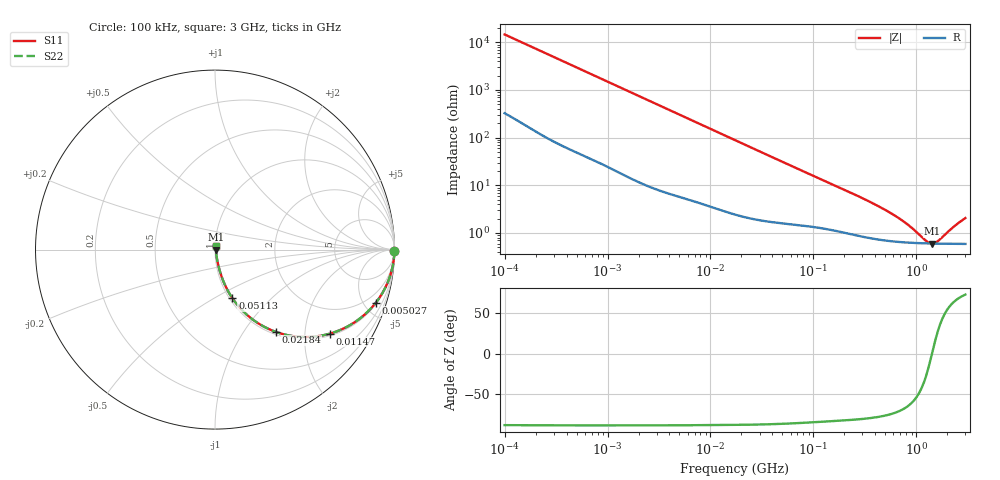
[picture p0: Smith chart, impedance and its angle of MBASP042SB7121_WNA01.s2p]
! MBASP042SB7121_WNA01  S-PARAMETER MODEL  ( Standard Model )
! Model Generated by TAIYO YUDEN Corporation (https://www.yuden.co.jp/en/)
! Version 1.0
! TAIYO YUDEN Control No. 250312
! Copyright(c) 2025 TAIYO YUDEN CO.,LTD. All Rights Reserved.
! Product Description (link to TY-COMPAS)
! https://ds.yuden.co.jp/TYCOMPAS/or/detail?pn=MBASP042SB7121KWNA01&u=M
! Products Name : Multilayer Ceramic Capacitors
! Characteristics :
!  Capacitance : 120 [pF] , Rated Voltage : 2.5 [V] , TCC : X7R
!  Case Size : 0.4 x 0.2 / 0.016 x 0.008 [mm/inch] , Thickness : 0.2 / 0.008 [mm/inch]
!  (Conditions: Temperature = 25 [degC] , DC Bias Voltage = 0 [V])
! External Node Assignments :
!  1  o---| |---o  2
! GND o---------o GND
! Frequency Range : 100kHz  -  3GHz  [ 401 STEP ]
# MHZ S RI R 50
! Freq[MHz].  S11 Real  S11 Imag  S21 Real  S21 Imag  S12 Real  S12 Imag  S22 Real  S22 Imag
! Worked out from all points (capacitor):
!   401 points, 100 kHz to 3 GHz, reference 50 ohm
!   read as one part in series: C = 108 pF near 105.3 kHz
!   lowest |Z| = 602 mohm at 1.421 GHz (marker M1)
!   series resonance near 1.421 GHz, so ESL is about 120 pH
!   S11 on the Smith chart (normalised r, x): 100 kHz: open; 5.027 MHz: 1.11, -6.04; 11.47 MHz: 1.06, -2.67; 21.84 MHz: 1.04, -1.41; 51.13 MHz: 1.03, -0.61; 3 GHz: 1.01, +0.04
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0.1  0.9998 -0.00684  0.000199 0.00684  0.000199 0.00684  0.9998 -0.00684
0.562235  0.998 -0.0376  0.00204 0.0376  0.00204 0.0376  0.998 -0.0376
1.458987  0.9892 -0.0958  0.0108 0.0958  0.0108 0.0958  0.9892 -0.0958
3.161081  0.9552 -0.1988  0.0448 0.1988  0.0448 0.1988  0.9552 -0.1988
5.026967  0.8969 -0.2949  0.1031 0.2949  0.1031 0.2949  0.8969 -0.2949
7.592607  0.7966 -0.3919  0.2034 0.3919  0.2034 0.3919  0.7966 -0.3919
11.46769  0.6383 -0.4686  0.3617 0.4686  0.3617 0.4686  0.6383 -0.4686
17.7727  0.4311 -0.4816  0.5689 0.4816  0.5689 0.4816  0.4311 -0.4816
21.84217  0.3378 -0.4581  0.6622 0.4581  0.6622 0.4581  0.3378 -0.4581
32.98988  0.1899 -0.3736  0.8101 0.3736  0.8101 0.3736  0.1899 -0.3736
51.12795  0.0966 -0.2706  0.9034 0.2706  0.9034 0.2706  0.0966 -0.2706
97.38194  0.0379 -0.1537  0.9621 0.1537  0.9621 0.1537  0.0379 -0.1537
158.9065  0.0208 -0.0974  0.9792 0.0974  0.9792 0.0974  0.0208 -0.0974
287.4592  0.0115 -0.0545  0.9885 0.0545  0.9885 0.0545  0.0115 -0.0545
547.5153  0.00742 -0.026  0.9926 0.026  0.9926 0.026  0.00742 -0.026
826.9535  0.00644 -0.0135  0.9936 0.0135  0.9936 0.0135  0.00644 -0.0135
1249.01  0.00603 -0.00307  0.994 0.00307  0.994 0.00307  0.00603 -0.00307
1420.79  0.00598 1.41e-06  0.994 -1.41e-06  0.994 -1.41e-06  0.00598 1.41e-06
1495.945  0.00597 0.00123  0.994 -0.00123  0.994 -0.00123  0.00597 0.00123
1616.196  0.00596 0.00308  0.994 -0.00308  0.994 -0.00308  0.00596 0.00308
2378.954  0.00605 0.0128  0.9939 -0.0128  0.9939 -0.0128  0.00605 0.0128
3000  0.00625 0.0195  0.9937 -0.0195  0.9937 -0.0195  0.00625 0.0195
